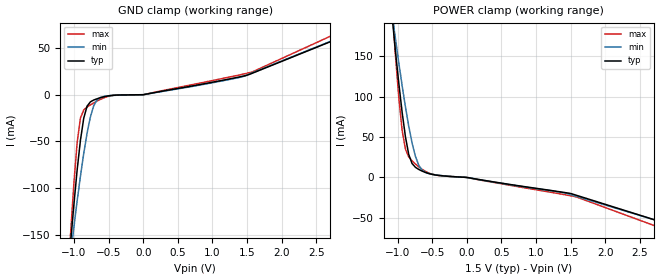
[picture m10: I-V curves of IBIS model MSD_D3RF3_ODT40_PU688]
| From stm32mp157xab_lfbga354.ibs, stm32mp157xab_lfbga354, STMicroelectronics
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[Model] MSD_D3RF3_ODT40_PU688
Model_type   Input
C_comp 2.345pF   2.303pF   2.424pF
Vinh = 925.000mV
Vinl = 575.000mV
[Temperature Range]   25.000   125.000   -40.000
[Voltage Range]   1.500V   1.425V   1.575V
[GND Clamp Reference]   0.00V   0.00V   0.00V
[POWER Clamp Reference]   1.500V   1.425V   1.575V
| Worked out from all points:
|   GND clamp passes 1 mA (typ) near -0.48 V on its own axis
|   POWER clamp passes 1 mA (typ) near -0.21 V on its own axis
[GND Clamp]
-1.48V    -590mA     -457.6mA   -789.2mA
-1.05V    -159.5mA   -171.9mA   -149.8mA
-1.002V   -118.1mA   -142.4mA   -95.35mA
-954.6mV  -80.7mA    -114mA     -51.35mA
-906.8mV  -48.8mA    -87.23mA   -25.01mA
-859.1mV  -25.08mA   -62.77mA   -16.32mA
-763.6mV  -7.686mA   -23.95mA   -10.92mA
-715.9mV  -5.73mA    -11.97mA   -8.8mA
-620.5mV  -3.268mA   -2.998mA   -5.048mA
900nV     12.82nA    11.99nA    14.85nA
1.575V    23.02mA    23.47mA    24.42mA
2.959V    64.49mA    64.89mA    71.4mA
[Power Clamp]
-1.459V   583.6mA    459.3mA    773.1mA
-1.077V   198.1mA    201.7mA    208.5mA
-1.03V    155.6mA    171.3mA    150.4mA
-981.8mV  116.3mA    141.7mA    98.58mA
-934.1mV  80.64mA    113.5mA    58.29mA
-886.4mV  50.27mA    87.28mA    35.01mA
-838.6mV  28.38mA    63.48mA    25.42mA
-790.9mV  17.2mA     42.85mA    20.53mA
-695.5mV  9.92mA     15.31mA    13.16mA
-504.6mV  3.8mA      3.907mA    4.021mA
1.548V    -21.2mA    -22.49mA   -23.53mA
2.98V     -59.72mA   -59.51mA   -68.23mA
